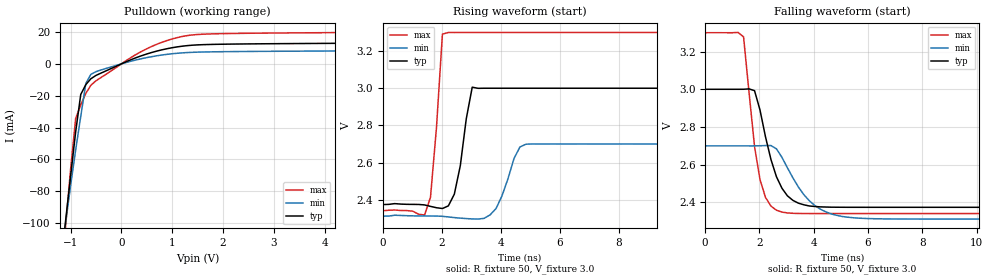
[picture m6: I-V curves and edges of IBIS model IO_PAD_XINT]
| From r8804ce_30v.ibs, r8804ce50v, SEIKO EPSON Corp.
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[Model]   IO_PAD_XINT
Model_type Open_drain
Enable Active-High
Polarity Non-Inverting
Vref=3.3
Vmeas=1.50
Rref=5000
C_comp   2.5p   2.0p   3.0p
[Temperature Range] 25   105   -40
[Voltage Range]   3.0   2.7   3.3
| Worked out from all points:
|   slope of the pulldown table from 0 to 0.45 V, typ, clamps not added: 79 ohm
|   falling waveform, R_fixture 50, V_fixture 3.0: 20-80 % time 707ps typ, 1.1ns min, 476ps max; typ from 3 V to 2.37 V
|   rising waveform, R_fixture 50, V_fixture 3.0: 20-80 % time 360ps typ, 502ps min, 266ps max; typ from 2.37 V to 3 V
[Pulldown]
-3V       -702.1mA   -577.4mA   -866.5mA
-1.1V     -99.04mA   -100.3mA   -102.6mA
-900mV    -42.59mA   -53.98mA   -34.23mA
-800mV    -19.2mA    -32.95mA   -25.77mA
-700mV    -13.01mA   -12.25mA   -18.5mA
-600mV    -9.326mA   -6.551mA   -13.4mA
-500mV    -7.242mA   -4.883mA   -10.62mA
500mV     6.223mA    3.955mA    9.514mA
900mV     9.547mA    6.005mA    14.7mA
1.3V      11.49mA    7.126mA    17.8mA
5V        13.19mA    8.301mA    20.03mA
6V        14.3mA     9.054mA    21.64mA
[Falling Waveform]
R_fixture=50
V_fixture=3.0
V_fixture_min=2.7
V_fixture_max=3.3
0s        3V         2.7V       3.3V
1.414ns   3V         2.7V       3.278V
1.818ns   2.993V     2.7V       2.697V
2.02ns    2.89V      2.7V       2.521V
2.424ns   2.627V     2.701V     2.38V
2.828ns   2.475V     2.639V     2.349V
3.232ns   2.411V     2.53V      2.342V
3.838ns   2.381V     2.409V     2.341V
5.051ns   2.374V     2.325V     2.341V
20ns      2.374V     2.312V     2.341V
[Rising Waveform]
R_fixture=50
V_fixture=3.0
V_fixture_min=2.7
V_fixture_max=3.3
0s        2.374V     2.312V     2.341V
1.414ns   2.372V     2.313V     2.318V
1.616ns   2.364V     2.313V     2.414V
1.818ns   2.357V     2.312V     2.787V
2.02ns    2.353V     2.311V     3.291V
2.424ns   2.43V      2.304V     3.3V
3.03ns    3.006V     2.297V     3.3V
3.838ns   3V         2.353V     3.3V
4.848ns   3V         2.699V     3.3V
20ns      3V         2.7V       3.3V
[Ramp]
R_load=50
dV/dt_r   3.755E-1/3.231E-10   2.328E-1/4.879E-10   5.754E-1/2.188E-10
dV/dt_f   3.755E-1/6.993E-10   2.329E-1/1.093E-9   5.754E-1/4.583E-10
|[End   IO_PAD_XINT
